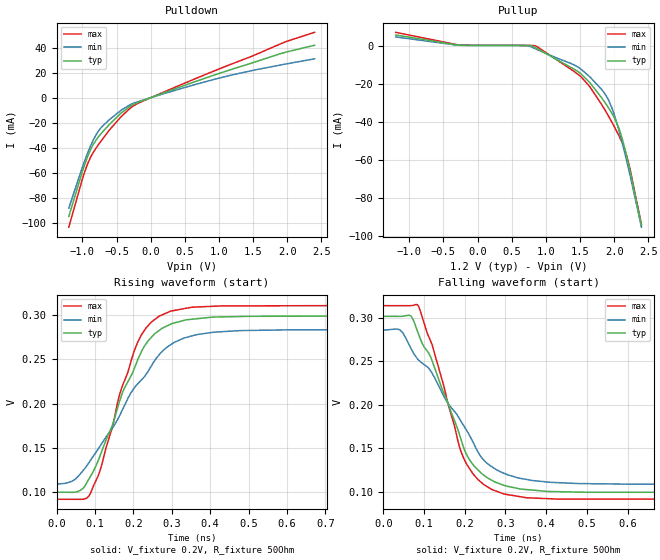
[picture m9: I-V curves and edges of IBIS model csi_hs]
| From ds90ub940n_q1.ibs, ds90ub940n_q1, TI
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|   Model
[Model]   csi_hs
Model_type   Output
Polarity   Non-Inverting
Vmeas = 0.2
Vref = 0.2
Cref = 1pF
Rref = 50
|   typ   min   max
C_comp   0.31pF   0.27pF   0.33pF
[Voltage Range]   1.2   1.14   1.26
[Temperature Range]   27   105   -40
[Pullup Reference]   1.2   1.14   1.26
[Pulldown Reference]   0   0   -0
[Power Clamp Reference]   1.2   1.14   1.26
[GND Clamp Reference]   0   0   0
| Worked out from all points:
|   slope of the pulldown table from 0 to 0.18 V, typ, clamps not added: 49.8 ohm
|   falling waveform, V_fixture 0.2V, R_fixture 50Ohm: 20-80 % time 99.1ps typ, 146ps min, 80.6ps max; typ from 0.302 V to 0.1 V
|   rising waveform, V_fixture 0.2V, R_fixture 50Ohm: 20-80 % time 110ps typ, 155ps min, 89.2ps max; typ from 0.1 V to 0.3 V
[Pulldown]
|   Voltage   I(typ)   I(min)   I(max)
-1.2V     -94.7mA    -88.08mA   -103.3mA
-984mV    -56.03mA   -52.85mA   -61.94mA
-912mV    -45.32mA   -42.52mA   -51.15mA
-847.2mV  -37.79mA   -34.37mA   -44.13mA
-789.6mV  -32.94mA   -28.53mA   -39.31mA
-721.2mV  -28.25mA   -23.55mA   -34.05mA
-433.2mV  -12.22mA   -9.959mA   -15.07mA
-300mV    -6.746mA   -5.538mA   -8.335mA
-98.4mV   -1.989mA   -1.655mA   -2.335mA
1.061V    20.41mA    16.43mA    24.21mA
2V        36.64mA    27.1mA     45.12mA
2.4V      41.86mA    31.02mA    52.16mA
[Pullup]
|   Voltage   I(typ)   I(min)   I(max)
-1.2V     5.659mA    4.637mA    7.061mA
-300mV    410.1uA    316.5uA    570.2uA
708mV     134.2uA    84.01uA    185.8uA
841.2mV   -864.8uA   -1.486mA   -9.963uA
1.514V    -14.72mA   -12.28mA   -16.26mA
1.655V    -19.86mA   -16.75mA   -22.1mA
1.838V    -28.43mA   -23.93mA   -32.14mA
1.975V    -36mA      -33.4mA    -40.71mA
2.076V    -44.01mA   -45.21mA   -47.68mA
2.177V    -57.04mA   -59.42mA   -57.04mA
2.234V    -66mA      -68.2mA    -65.03mA
2.4V      -94.45mA   -95.28mA   -93.95mA
[Ramp]
R_load = 50
|   typ   min   max
dV/dt_r   0.120128/1.09909e-10   0.105158/1.55131e-10   0.132241/8.91306e-11
dV/dt_f   0.121154/9.91213e-11   0.106035/1.45577e-10   0.133302/8.06469e-11
[Falling Waveform]
V_fixture = 0.2V
V_fixture_min = 0.2V
V_fixture_max = 0.2V
R_fixture = 50Ohm
C_fixture = 0F
|   Time   V(typ)   V(min)   V(max)
0s        301.6mV    285.7mV    313.8mV
39.66ps   301.5mV    286.3mV    313.8mV
68.48ps   301.5mV    264mV      313.9mV
83.75ps   284.5mV    252.8mV    314.8mV
119.5ps   250.8mV    236.6mV    269.5mV
196.8ps   151.5mV    176.5mV    139.4mV
244.1ps   120.4mV    137.9mV    109.7mV
297.2ps   107.6mV    121.4mV    97.68mV
480.2ps   99.97mV    109.8mV    91.97mV
1.7ns     99.63mV    109mV      91.67mV
[Rising Waveform]
V_fixture = 0.2V
V_fixture_min = 0.2V
V_fixture_max = 0.2V
R_fixture = 50Ohm
C_fixture = 0F
|   Time   V(typ)   V(min)   V(max)
0s        99.63mV    108.9mV    91.67mV
53.48ps   100mV      116.3mV    91.61mV
87.33ps   116.9mV    135mV      97.43mV
115.9ps   143.8mV    153.5mV    127.8mV
163.6ps   202mV      185.8mV    209.1mV
210.8ps   248.8mV    222mV      269mV
240.1ps   271.8mV    237.6mV    288.9mV
297.2ps   289.8mV    266.5mV    304.6mV
480.2ps   298.5mV    282.6mV    310.5mV
1.7ns     299.8mV    284.1mV    312.1mV
